FUNCTION_BLOCK RANGEJD
VAR_INPUT
	ENABLE:BOOL;
	SV:LREAL;
	PV:LREAL;
	RANGE_ALARM_H:LREAL;
	RANGE_ALARM_L:LREAL;
	RANGE_WARNING_H:LREAL;
	RANGE_WARNING_L:LREAL;
	TIME_ALARM:LREAL;
	TIME_WARNING:LREAL;
	
END_VAR
VAR_OUTPUT
	ALARM:BOOL;
	WARNING:BOOL;
END_VAR
VAR
	TON_ALARM:TON;
	TON_WARNING:TON;
	STATUS_ALARM:BOOL;
	STATUS_WARNING:BOOL;
END_VAR

IF ENABLE
	THEN	
	IF PV	>=	(SV+RANGE_ALARM_H) OR 	PV	<=	(SV-RANGE_ALARM_L)
		THEN	STATUS_ALARM:=TRUE;
		ELSE	STATUS_ALARM:=FALSE;
	END_IF		
	
	IF PV	>=	(SV+RANGE_WARNING_H) OR 	PV	<=	(SV-RANGE_WARNING_L)
		THEN	STATUS_WARNING:=TRUE;
		ELSE	STATUS_WARNING:=FALSE;
	END_IF	
	
	TON_ALARM(IN:=STATUS_ALARM , PT:= LREAL_TO_TIME(TIME_ALARM)*1000, Q=> , ET=> );		
	IF TON_ALARM.Q		
		THEN	
		ALARM:=TRUE;	
		ELSE	
		ALARM:=FALSE;	
	END_IF	
	
	TON_WARNING(IN:=STATUS_WARNING , PT:= LREAL_TO_TIME(TIME_WARNING)*1000, Q=> , ET=> );		
	IF TON_WARNING.Q		
		THEN	
		WARNING:=TRUE;	
		ELSE	
		WARNING:=FALSE;	
	END_IF	

	ELSE
		STATUS_ALARM:=FALSE;
		STATUS_WARNING:=FALSE;
		ALARM:=FALSE;
		WARNING:=FALSE;	
END_IF
	
	IF NOT ENABLE
	THEN
	STATUS_ALARM:=FALSE;
	STATUS_WARNING:=FALSE;
	END_IF

END_FUNCTION_BLOCK
